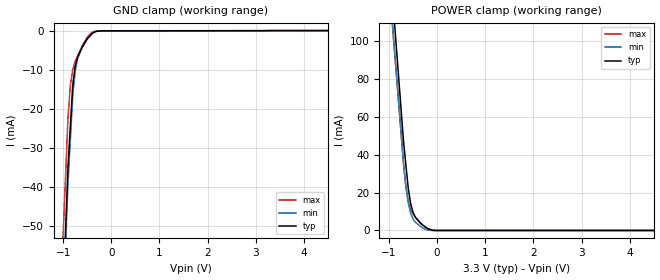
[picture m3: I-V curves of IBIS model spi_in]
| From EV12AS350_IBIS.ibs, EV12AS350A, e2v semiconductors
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[Model] spi_in
Model_type Input
Vinl = 1.15500V
Vinh = 2.14500V
C_comp 463.000fF 423.000fF 483.000fF
| variable typ   min   max
[Voltage Range] 3.30000V 3.20000V 3.40000V
[POWER Clamp Reference] 3.30000V 3.20000V 3.40000V
[GND Clamp Reference] 0.00000V 0.00000V 0.00000V
[Temperature Range]   25   110   -40
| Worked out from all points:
|   GND clamp passes 1 mA (typ) near -0.42 V on its own axis
|   POWER clamp passes 1 mA (typ) near -0.19 V on its own axis
[GND Clamp]
-3.3V     -812mA     -788.4mA   -738.5mA
-900mV    -34.87mA   -39.32mA   -22.28mA
-850mV    -24.34mA   -27.96mA   -13.9mA
-800mV    -13.81mA   -16.61mA   -9.923mA
-750mV    -9.089mA   -10.3mA    -7.806mA
-700mV    -6.718mA   -7.135mA   -6.452mA
-600mV    -4.056mA   -4.17mA    -3.743mA
-500mV    -2.042mA   -2.159mA   -1.697mA
-450mV    -1.367mA   -1.473mA   -956.3uA
-350mV    -311.9uA   -376.9uA   -157.5uA
-150mV    -29.78uA   -42.24uA   -8.053uA
6.6V      32.17uA    39.54uA    26.35uA
[POWER Clamp]
-3.3V     918.7mA    866mA      865.5mA
-800mV    81.35mA    67.97mA    68.15mA
-700mV    47.86mA    36.05mA    36.26mA
-650mV    35.12mA    23.36mA    23.58mA
-600mV    22.37mA    14.65mA    15.44mA
-550mV    14.23mA    8.998mA    10.97mA
-500mV    9.486mA    6.122mA    8.59mA
-450mV    6.963mA    4.311mA    7.001mA
-300mV    2.881mA    1.247mA    2.848mA
-200mV    1.095mA    206.1uA    899.7uA
-50mV     0A         0A         47.36uA
6.6V      0A         0A         0A
